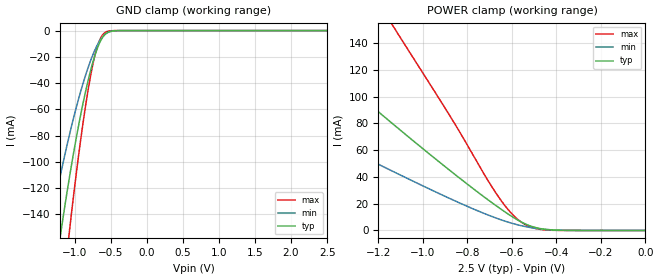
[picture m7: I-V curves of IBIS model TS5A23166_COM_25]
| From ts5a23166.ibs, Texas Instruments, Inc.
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[Model]   TS5A23166_COM_25
Model_type  Terminator
| variable   typ   min   max
C_comp   18.54pF   17.67pF   20.10pF
| C_tri-state   18.54pF   17.67pF   20.10pF
[Temperature Range]   40   100   -40
| Ambient temperature   25   85   -40
[Voltage range]   2.5   2.3   2.7
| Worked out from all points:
|   GND clamp passes 1 mA (typ) near -0.53 V on its own axis
|   POWER clamp passes 1 mA (typ) near -0.46 V on its own axis
[GND Clamp]
| TS5A23166_COM_25
|   Voltage   I(typ)   I(min)   I(max)
-2.5V     -809mA     -586.1mA   -1.101A
-1.355V   -218.6mA   -154mA     -306.7mA
-1.205V   -159.3mA   -112.4mA   -221.7mA
-1.18V    -150mA     -106mA     -208.2mA
-1.085V   -116.4mA   -82.63mA   -159.5mA
-1.065V   -109.7mA   -77.98mA   -149.8mA
-910mV    -62.69mA   -45.32mA   -81.01mA
-780mV    -30.87mA   -23.18mA   -34.99mA
-675mV    -12.18mA   -9.988mA   -10.57mA
-570mV    -2.51mA    -2.515mA   -1.18mA
-395mV    -34.12uA   -61.53uA   -3.164uA
2.5V      769.9pA    2.263uA    62.85pA
[POWER Clamp]
| TS5A23166_COM_25
|   Voltage   I(typ)   I(min)   I(max)
-2.5V     314mA      183.7mA    595.5mA
-2.205V   254.2mA    147.8mA    483.5mA
-1.62V    150.4mA    85.9mA     288.6mA
-1.155V   82.36mA    45.78mA    158.3mA
-1.105V   75.43mA    41.72mA    145mA
-880mV    45mA       23.94mA    85.96mA
-685mV    20.17mA    10.13mA    31.28mA
-625mV    13.16mA    6.651mA    17.2mA
-565mV    6.968mA    3.842mA    7.092mA
-515mV    3.24mA     2.138mA    2.477mA
-450mV    857.4uA    792.8uA    414.9uA
-31.15fV  769.9pA    6.273nA    80.69pA
